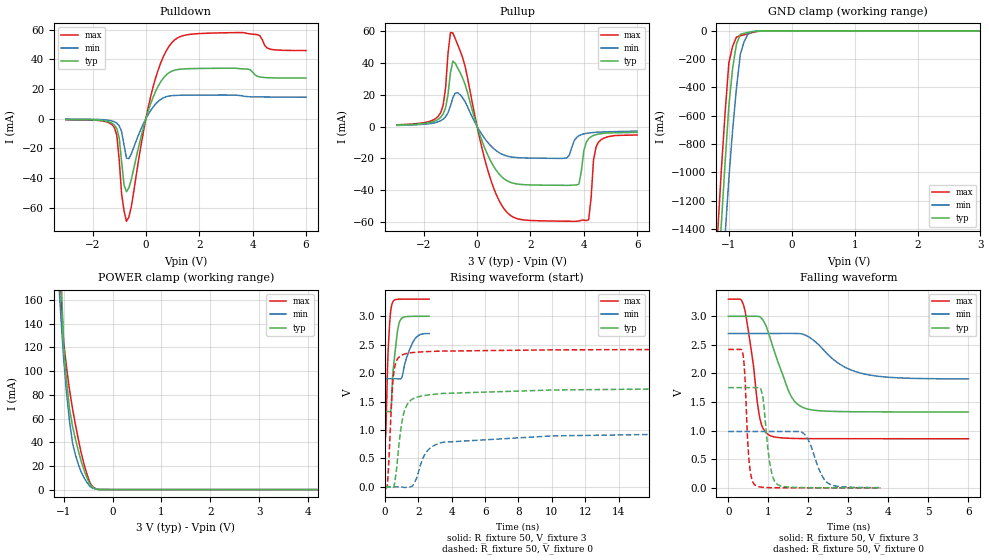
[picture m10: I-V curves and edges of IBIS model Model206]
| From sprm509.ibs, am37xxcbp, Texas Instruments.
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| Model based on original model for BQMMC1833DVHYPBFZLP18_SSCHH
|   Sub model CHH_SPEEDCTRL0_PD1_3
[model]   Model206
|[Input Load]   PD
|[Output Drive] SC0
|Voltage   3V
|Mode   I/O
Model_type   I/O
Polarity   Non-Inverting
Enable   Active-Low
Vinl =  0.9
Vinh =  2.1
Cref =  15pF
Rref =  100.0000M
Vref =  0V
Vmeas =  1.5
C_comp   5.193555p   4.924275p   5.205586p
[Model Spec]
Vinl   0.9   0.81   0.99
Vinh   2.1   1.89   2.31
[Temperature Range]   25   125   -40
[Voltage Range]   3   2.7   3.3
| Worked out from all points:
|   slope of the pulldown table from 0 to 0.45 V, typ, clamps not added: 20.8 ohm
|   slope of the pullup table from 0 to 0.45 V, typ, clamps not added: 22.8 ohm
|   GND clamp passes 1 mA (typ) near -0.51 V on its own axis
|   POWER clamp passes 1 mA (typ) near -0.36 V on its own axis
|   rising waveform, R_fixture 50, V_fixture 3: 20-80 % time 304ps typ, 548ps min, 180ps max; typ from 1.32 V to 3 V
|   rising waveform, R_fixture 50, V_fixture 0: 20-80 % time 550ps typ, 1.52ns min, 266ps max; typ from 0 V to 1.75 V
|   falling waveform, R_fixture 50, V_fixture 3: 20-80 % time 504ps typ, 861ps min, 271ps max; typ from 3 V to 1.33 V
|   falling waveform, R_fixture 50, V_fixture 0: 20-80 % time 166ps typ, 320ps min, 102ps max; typ from 1.75 V to 0.001 V
[POWER_clamp]
-3V       3.885A     1.82A      4.094A
-1.121V   269.1mA    190mA      236.5mA
-1.061V   190mA      149.2mA    170.5mA
-1V       123.2mA    111mA      124.9mA
-939.4mV  91.3mA     81.53mA    102.9mA
-878.8mV  68.12mA    57.7mA     84.07mA
-818.2mV  53.62mA    39.48mA    68.5mA
-697mV    32.46mA    21mA       42.06mA
-575.8mV  15.74mA    9.608mA    20.45mA
-454.5mV  4.037mA    2.416mA    5.101mA
-393.9mV  1.738mA    1.086mA    2.148mA
6V        0A         0A         0A
[Pulldown]
-3V       -605.8uA   -178.5uA   -753.3uA
-1.182V   -4.21mA    -2.052mA   -5.965mA
-1.091V   -6.698mA   -2.971mA   -10.98mA
-1V       -12.89mA   -4.735mA   -27.71mA
-909.1mV  -29.13mA   -8.689mA   -50.98mA
-727.3mV  -49.28mA   -26.6mA    -69.24mA
-545.5mV  -40.99mA   -23.62mA   -59.29mA
272.7mV   14.65mA    7.964mA    21.68mA
1V        32.33mA    15.62mA    51.9mA
3.636V    33.67mA    15.32mA    58.15mA
4.636V    27.65mA    14.67mA    47.11mA
6V        27.45mA    14.53mA    46.04mA
[Pullup]
-3V       909.3uA    688uA      1.095mA
-1.364V   5.79mA     3.639mA    8.811mA
-1V       33.75mA    12.82mA    59.02mA
-545.5mV  30.59mA    18.14mA    43.38mA
545.5mV   -22.87mA   -12.71mA   -35.18mA
1.364V    -35.67mA   -19.33mA   -57.01mA
3.364V    -36.98mA   -19.72mA   -59.51mA
3.818V    -36.13mA   -5.779mA   -59.33mA
4.182V    -7.586mA   -4.088mA   -58.55mA
4.364V    -5.632mA   -3.758mA   -21mA
4.545V    -4.785mA   -3.538mA   -9.97mA
6V        -3.687mA   -2.885mA   -5.329mA
[GND_clamp]
-3V       -17.89A    -17.26A    -17.77A
-1.182V   -1.843A    -2.308A    -1.459A
-1.121V   -1.377A    -1.871A    -995.4mA
-1.061V   -939mA     -1.45A     -584.5mA
-1V       -529.9mA   -1.045A    -225.8mA
-939.4mV  -261.2mA   -697mA     -108mA
-878.8mV  -92.98mA   -404.2mA   -44.13mA
-818.2mV  -25.12mA   -166.6mA   -34.22mA
-757.6mV  -17.49mA   -76.74mA   -28.22mA
-697mV    -11.17mA   -23.3mA    -21.17mA
-575.8mV  -3.102mA   -3.059mA   -6.967mA
3V        36.99uA    104.7uA    51.93uA
[Ramp]
dV/dt_f   1.005749/0.5024452n  0.4796256/0.8718953n   1.464851/0.2696084n
dV/dt_r   1.060556/0.5437606n  0.5963999/1.532923n   1.462407/0.2656033n
R_load = 50
[Rising Waveform]
R_fixture = 50
V_fixture = 3
V_fixture_min = 2.7
V_fixture_max = 3.3
0s        1.324V     1.901V     856.6mV
44ps      1.324V     1.901V     944.8mV
154ps     1.324V     1.901V     2.157V
198ps     1.324V     1.901V     2.467V
352ps     1.355V     1.901V     3.117V
418ps     1.718V     1.901V     3.214V
726ps     2.692V     1.9V       3.296V
924ps     2.934V     1.899V     3.298V
1.738ns   2.997V     2.576V     3.299V
2.64ns    2.998V     2.694V     3.299V
[Rising Waveform]
R_fixture = 50
V_fixture = 0
V_fixture_min = 0
V_fixture_max = 0
0s        1.081uV    2.723uV    -1.075mV
132ps     1.906uV    2.704uV    8.126mV
440ps     -14.39mV   3.117uV    1.733V
616ps     152.9mV    -17.7uV    2.158V
1.21ns    1.375V     -9.545mV   2.339V
1.65ns    1.544V     17.41mV    2.36V
2.332ns   1.604V     542.5mV    2.375V
3.454ns   1.642V     784.1mV    2.386V
16.68ns   1.721V     923.8mV    2.414V
162.2ns   1.753V     980mV      2.42V
[Falling Waveform]
R_fixture = 50
V_fixture = 3
V_fixture_min = 2.7
V_fixture_max = 3.3
0s        2.999V     2.7V       3.299V
308ps     2.999V     2.7V       3.296V
396ps     2.999V     2.7V       3.162V
616ps     3V         2.7V       2.208V
792ps     2.989V     2.7V       1.209V
1.034ns   2.647V     2.7V       918.3mV
1.562ns   1.612V     2.7V       865.6mV
1.87ns    1.404V     2.686V     861.7mV
3.278ns   1.331V     2.012V     859.3mV
6.006ns   1.326V     1.906V     858.8mV
[Falling Waveform]
R_fixture = 50
V_fixture = 0
V_fixture_min = 0
V_fixture_max = 0
0s        1.753V     985.4mV    2.42V
352ps     1.753V     985.4mV    2.385V
528ps     1.753V     985.4mV    409.7mV
660ps     1.754V     985.4mV    55.1mV
858ps     1.617V     985.4mV    10.24mV
1.034ns   445.2mV    985.4mV    4.12mV
1.232ns   58.03mV    985.4mV    2.113mV
1.936ns   4.838mV    915.2mV    685.3uV
2.508ns   2.363mV    75.41mV    430.1uV
3.806ns   1.182mV    5.523mV    228.5uV
